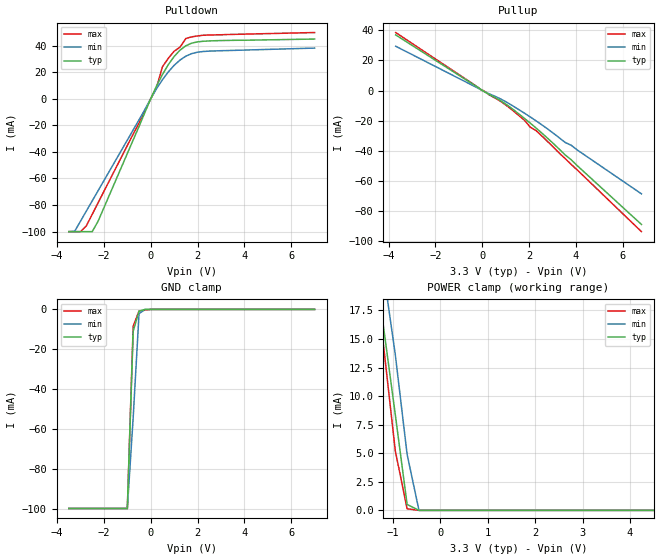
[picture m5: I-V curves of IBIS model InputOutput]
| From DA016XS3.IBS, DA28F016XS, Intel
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|**********************Input Output Model**********************************
[Model]   InputOutput
Model_type   I/O
|   for DQ[15:0]
Vinl = 0.8V
Vinh = 2.0V
| Variable   typ   min   max
C_comp   9.61p   NA   11.6p
[Voltage Range]   3.3V   3.0V   3.6V
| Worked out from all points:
|   slope of the pulldown table from 0 to 0.495 V, typ, clamps not added: 27.5 ohm
|   slope of the pullup table from 0 to 0.495 V, typ, clamps not added: 116 ohm
|   GND clamp passes 1 mA (typ) near -0.50 V on its own axis
|   POWER clamp passes 1 mA (typ) near -0.72 V on its own axis
[Pulldown]
| [Pullup] and [Pulldown] IV curves include only the current through
| the channels of output driver transistors when outputs are enabled
| with OE# = VIL.  Although the output driver transistors have np and
| pn diodes inherently created by CMOS IC fabrication between the
| drain and bulk of n-channel and p-channel CMOS transistors,
| the current through these junction diodes is not included in
| [Pullup] or [Pulldown].  Instead that drain/bulk diode current is
| included in the [POWER_clamp] or [GND_clamp] sections, which are
| not dependent on the state of OE# or output data value.
|Voltage  I(typ)   I(min)   I(max)
-3.5V     -100mA     -100mA     -100mA
-3.25V    -100mA     -99.73mA   -100mA
-3V       -100mA     -92.1mA    -100mA
-2.75V    -100mA     -84.48mA   -95.58mA
-2.5V     -100mA     -76.85mA   -86.95mA
-2.25V    -92.2mA    -69.23mA   -78.33mA
250mV     9.634mA    7.57mA     8.69mA
500mV     18.18mA    14.27mA    24.05mA
1V        31.79mA    25.13mA    35.73mA
1.5V      39.84mA    32.02mA    45.29mA
2.5V      43.48mA    35.83mA    47.93mA
7V        44.9mA     38.1mA     49.8mA
[GND_clamp]
| [POWER_clamp] and [GND_clamp] IV curves describe ESD protection
| circuits PLUS some np and pn diodes which exist between the
| drain and bulk of n-channel and p-channel CMOS transistors.
| These drain/bulk diodes are inherent in CMOS IC fabrication,
| and are visible on the node of the I/O pin at all times.
| Even the drain/bulk diodes of output driver [Pullup] and [Powerdown]
| transistors are included in [POWER_clamp] or [GND_clamp], because
| these diodes contribute to I/O pin current even when the
| chip outputs are tristated by OE# = VIH.
| For example, when V forced on the I/O pin is large, we are
| forward biasing the pn diode at the drain/bulk interface in the
| p-channel pullup transistor.  Similarly, when V forced on the
| I/O pin is sufficiently negative with respect to the substrate
| ground, we are forward biasing the np diode at the drain/bulk
| interface in the n-channel pulldown transistor.  The effects
| of these diodes are included in [POWER_clamp] or [GND_clamp].
|Voltage  I(typ)   I(min)   I(max)
-3.5V     -99.93mA   -99.94mA   -99.95mA
-1V       -99.93mA   -99.94mA   -99.94mA
-750mV    -10.94mA   -54.25mA   -8.45mA
-500mV    -899.5uA   -2.128mA   -770uA
-250mV    0A         -55.09uA   -410uA
0V        0A         0A         0A
7V        0A         0A         0A
[Pullup]
| (Voltages for [Pullup] and [POWER_clamp] are specified with
| negative respect to Vcc.  Reference the IBIS documentation
| for more information regarding Vtable = Vcc - Voutput.
| This method keeps -Vds constant for the values in all three
| columns across a line of the table.
| [Pullup] and [Pulldown] IV curves include only the current through
| the channels of output driver transistors when outputs are enabled
| with OE# = VIL.  Although the output driver transistors have np and
| pn diodes inherently created by CMOS IC fabrication between the
| drain and bulk of n-channel and p-channel CMOS transistors,
| the current through these junction diodes is not included in
| [Pullup] or [Pulldown].  Instead that drain/bulk diode current is
| included in the [POWER_clamp] or [GND_clamp] sections, which are
| not dependent on the state of OE# or output data value.
|Voltage  I(typ)   I(min)   I(max)
-3.7V     36.83mA    29.33mA    38.41mA
0V        0A         0A         0A
50mV      -453.2uA   -371.9uA   -14uA
800mV     -6.86mA    -5.713mA   -7.322mA
1.3V      -12.37mA   -10.15mA   -13.21mA
1.8V      -18.46mA   -15.02mA   -19.71mA
2.05V     -21.63mA   -17.53mA   -24.3mA
2.3V      -24.89mA   -20.12mA   -26.59mA
2.55V     -28.29mA   -22.81mA   -30.22mA
3.55V     -42.81mA   -34.51mA   -45.23mA
3.8V      -45.92mA   -36.28mA   -49.01mA
6.8V      -88.76mA   -68.48mA   -93.52mA
[POWER_clamp]
| (Voltages for [Pullup] and [POWER_clamp] are specified with
| negative respect to Vcc.  Reference the IBIS documentation
| for more information regarding Vtable = Vcc - Voutput.
| This method keeps -Vds constant for the values in all three
| columns across a line of the table. For example, on the seventh
| line of the table below, Voltage = -2V on this 3.3V+-10% VCC model
| means Voutput with respect to ground is forced to about 5.3(typ),
| 5.0V (min), and 5.6V (max), and in all three cases -Vds = -2V.)
| [POWER_clamp] and [GND_clamp] IV curves describe ESD protection
| circuits PLUS some np and pn diodes which exist between the
| drain and bulk of n-channel and p-channel CMOS transistors.
| These drain/bulk diodes are inherent in CMOS IC fabrication,
| and are visible on the node of the I/O pin at all times.
| Even the drain/bulk diodes of output driver [Pullup] and [Pulldown]
| transistors are included in [POWER_clamp] or [GND_clamp], because
| these diodes contribute to I/O pin current even when the
| chip outputs are tristated by OE# = VIH.
| For example, when V forced on the I/O pin is large, we are
| forward biasing the pn diode at the drain/bulk interface in the
| p-channel pullup transistor.  Similarly, when V forced on the
| I/O pin is sufficiently negative with respect to the substrate
| ground, we are forward biasing the np diode at the drain/bulk
| interface in the n-channel pulldown transistor.  The effects
| of these diodes are included in [POWER_clamp] or [GND_clamp].
|Voltage  I(typ)   I(min)   I(max)
-3.7V     74.83mA    74.52mA    73.77mA
-1.45V    22.75mA    27.27mA    20mA
-1.2V     16.12mA    20.94mA    14.53mA
-950mV    8.403mA    13.65mA    5.23mA
-700mV    518uA      4.9mA      137uA
-450mV    0A         0A         0A
6.8V      0A         0A         0A
[Ramp]
| The DQ Ramp information is not provided at this time for the
| device but will be available in the future.  The table below
| is for the compatibility with some IBIS parsers.
| Variable   typ   min   max
 dV/dt_r   0V/0ns   0V/0ns   0V/0ns
 dV/dt_f   0V/0ns   0V/0ns   0V/0ns
